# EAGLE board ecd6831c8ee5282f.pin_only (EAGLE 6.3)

Size 20.32 x 17.78 mm. Coordinates in mm from the lower left corner, seen from the top.
Outline: 1.91,17.78 18.41,17.78 arc-90 20.32,15.88 20.32,1.91 arc-90 18.41,0 1.91,0 arc-90 0,1.91 0,15.88 arc-90 1.91,17.78
Copper layers (1*16): Top 0.035mm / dielectric 1.5mm / Bottom 0.035mm
Design rules "default": minimum track width 8mil, minimum drill 16mil, track to track 8mil, track to pad 8mil, pad to pad 8mil, via to via 8mil, smd to smd 8mil, copper to edge 10mil, drill to drill 8mil, minimum pad ring 10mil, minimum via ring 8mil, stop-mask expansion 4mil, vias tented up to drill 20mil, thermal gap 10mil
Holes 2.8 mm at 2.03,15.75 2.03,2.03 18.29,15.75 18.29,2.03

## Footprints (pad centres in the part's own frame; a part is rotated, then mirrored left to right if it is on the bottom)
C0805 = smd 1.3 x 1.5: 1 -0.85,0; 2 0.85,0
1X04-CLEANBIG = drill 1.016 pad 1.778: 1 -3.81,0; 2 -1.27,0; 3 1.27,0; 4 3.81,0
FIDUCIAL_1MM = smd 1 x 1: 1 0,0
MC14093B-TSSOP14 = smd 0.36 x 1.26: 1 -1.95,-2.925; 2 -1.3,-2.925; 3 -0.65,-2.925; 4 0,-2.925; 5 0.65,-2.925; 6 1.3,-2.925; 7 1.95,-2.925; 8 1.95,2.925; 9 1.3,2.925; 10 0.65,2.925; 11 0,2.925; 12 -0.65,2.925; 13 -1.3,2.925; 14 -1.95,2.925
CHIP-LED0805 = smd 1.2 x 1.2: A 0,-1.05; C 0,1.05
SOT23-BEC = smd 1 x 1.4: B -0.95,-1.1; C 0,1.1; E 0.95,-1.1
SOT23-WIDE = smd 1 x 1.2: 1 -0.95,-1; 2 0.95,-1; 3 0,1
R0805 = smd 1.3 x 1.5: 1 -0.95,0; 2 0.95,0
R0805' = smd 1.1 x 1.4: 1 -1,0; 2 1,0
B3F-40XX-ROUND = drill 1.194 pad 2.54: 1 -6.248,2.489; 2 6.248,2.489; 3 -6.248,-2.489; 4 6.248,-2.489 | hole 1.803: 0,-4.496; 0,4.496

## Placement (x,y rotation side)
C1  0.1uF  [C0805]  5.46,5.33 90 top
CN1  1X4-CLEANBIG  [1X04-CLEANBIG]  1.27,8.89 90 bottom
CN2  1X4-CLEANBIG  [1X04-CLEANBIG]  19.05,8.89 90 bottom
FID1  FIDUCIAL""  [FIDUCIAL_1MM]  17.27,4.32 0 top
FID2  FIDUCIAL""  [FIDUCIAL_1MM]  4.57,16.38 0 top
FID3  FIDUCIAL""  [FIDUCIAL_1MM]  3.3,4.45 0 top
IC1  4093DT  [MC14093B-TSSOP14]  10.16,8.89 0 top
LED  RED  [CHIP-LED0805]  10.16,2.29 0 top
Q1  2N2222  [SOT23-BEC]  15.24,11.3 90 top
Q2  POWER PFET  [SOT23-WIDE]  4.83,11.68 90 top
R1  1K  [R0805]  15.24,2.54 90 top
R2  100K  [R0805]  15.49,15.24 90 top
R3  100K  [R0805]  10.16,15.24 90 top
R4  1K  [R0805']  15.49,6.35 180 top
S1  [B3F-40XX-ROUND]  10.16,8.89 90 bottom
U$1  [ADAFRUIT_2.5MM]  11.3,15.24 0 bottom
U$2  [ADAFRUIT_2.5MM]  3.68,0.64 0 top

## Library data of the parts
C1 CN1 CN2 IC1 LED R4 S1 = adafruit
FID1-FID3 = microbuilder; BOM: EXCLUDE
Q1 = transistor
Q2 U$1 U$2 = microbuilder
R1-R3 = rcl

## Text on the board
bPlace: 3A Max | 3-14V | In | In | Out | Out | G | G | Off | Off | Mom. Powerswitch

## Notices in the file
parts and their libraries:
microbuilder: This work is placed in the public domain, and may be freely used for commercial and non-commercial work with the following conditions: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
